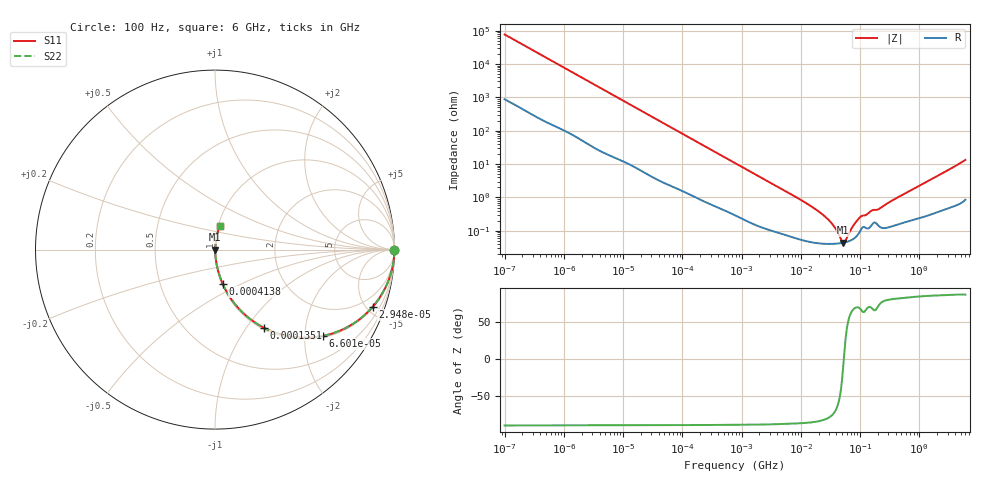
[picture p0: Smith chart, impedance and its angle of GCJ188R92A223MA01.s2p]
!Murata Part Number: GCJ188R92A223MA01
!These Parameters are Measured in Series Mode Connection
!Data Generated on Mar 13, 2026
!  o--ll--o
!Port1  Port2
!  o------o
!Operation Temp=25[degC], DC Bias Voltage=0[V]
!Freq. Start=100[Hz] Stop=6[GHz] 401[Steps]
# Hz S RI R 50
!Freq.(Hz) S11(Real) S11(Imag) S21(Real) S21(Imag) S12(Real) S12(Imag) S22(Real) S22(Imag)
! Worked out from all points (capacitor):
!   401 points, 100 Hz to 6 GHz, reference 50 ohm
!   read as one part in series: C = 20.7 nF near 109 Hz
!   lowest |Z| = 44.6 mohm at 52.11 MHz (marker M1)
!   series resonance near 53.17 MHz, so ESL is about 430 pH
!   S11 on the Smith chart (normalised r, x): 100 Hz: open; 29.48 kHz: 1.09, -5.45; 66 kHz: 1.04, -2.45; 135.1 kHz: 1.02, -1.21; 413.8 kHz: 1.01, -0.40; 6 GHz: 1.02, +0.27
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100  1 -0.0013  1.66e-05 0.0013  1.66e-05 0.0013  1 -0.0013
2008  0.999 -0.0255  0.00099 0.0255  0.00099 0.0255  0.999 -0.0255
9204  0.9851 -0.1139  0.0149 0.1139  0.0149 0.1139  0.9851 -0.1139
29482  0.8777 -0.3199  0.1223 0.3199  0.1223 0.3199  0.8777 -0.3199
40335  0.796 -0.395  0.204 0.395  0.204 0.395  0.796 -0.395
66005  0.5993 -0.4813  0.4007 0.4813  0.4007 0.4813  0.5993 -0.4813
135116  0.2718 -0.435  0.7282 0.435  0.7282 0.435  0.2718 -0.435
221108  0.1267 -0.3221  0.8733 0.3221  0.8733 0.3221  0.1267 -0.3221
413847  0.0428 -0.1908  0.9572 0.1908  0.9572 0.1908  0.0428 -0.1908
774597  0.0144 -0.1062  0.9856 0.1062  0.9856 0.1062  0.0144 -0.1062
2481164  0.00233 -0.0341  0.9977 0.0341  0.9977 0.0341  0.00233 -0.0341
1.555665e7  0.000476 -0.00517  0.9995 0.00517  0.9995 0.00517  0.000476 -0.00517
3.045065e7  0.000409 -0.00196  0.9996 0.00196  0.9996 0.00196  0.000409 -0.00196
5.211241e7  0.00044 -6.72e-05  0.9996 6.72e-05  0.9996 6.72e-05  0.00044 -6.72e-05
5.699437e7  0.000457 0.000236  0.9995 -0.000236  0.9995 -0.000236  0.000457 0.000236
7.797396e7  0.000579 0.00136  0.9994 -0.00136  0.9994 -0.00136  0.000579 0.00136
1.020051e8  0.00104 0.00242  0.999 -0.00242  0.999 -0.00242  0.00104 0.00242
1.596157e8  0.00156 0.00379  0.9984 -0.00379  0.9984 -0.00379  0.00156 0.00379
2.088084e8  0.00139 0.0043  0.9986 -0.0043  0.9986 -0.0043  0.00139 0.0043
3.124326e8  0.00134 0.00709  0.9987 -0.00709  0.9987 -0.00709  0.00134 0.00709
1.95892e9  0.00533 0.0423  0.9947 -0.0423  0.9947 -0.0423  0.00533 0.0423
6e9  0.0256 0.1289  0.9744 -0.1289  0.9744 -0.1289  0.0256 0.1289
